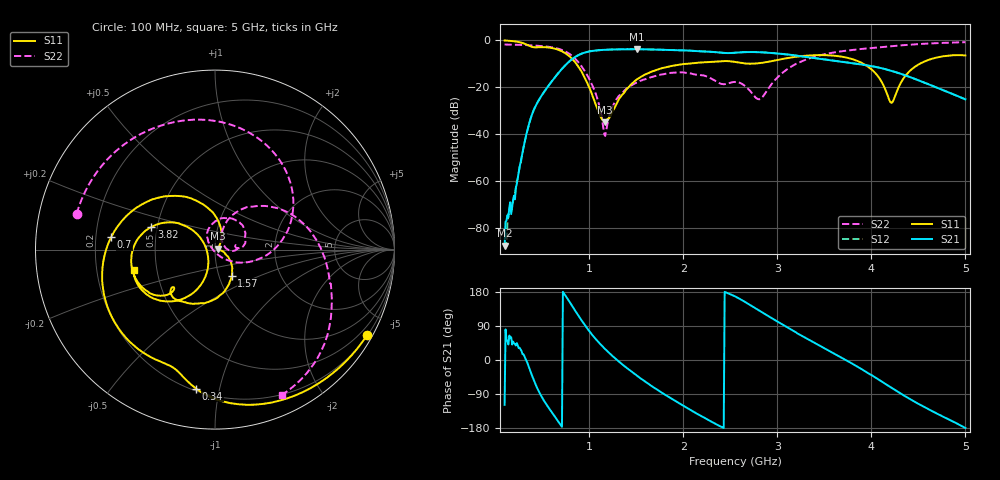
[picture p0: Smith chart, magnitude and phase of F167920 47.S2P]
!  2-Port S-parameters saved by WinCal
! VAR MeasName=S-Parameters (CALIBRATED_DATA) read from VNA (N5242A)
! VAR MeasDate=2016-11-22 9:57:49
! VAR NAME=F167920 47
! VAR FILENAME=F167920 47.S2P
! VAR DATE=2016-11-22 9:57:49
! VAR PHYS_PORTS=1,2
# Hz S DB R 50
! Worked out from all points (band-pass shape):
!   491 points, 100 MHz to 5 GHz, reference 50 ohm
!   highest |S21| = -3.95 dB at 1.51 GHz (marker M1); lowest = -87.6 dB at 100 MHz (marker M2)
!   |S21| within 3 dB of the highest: 863.3 MHz to 3.248 GHz (2.385 GHz wide, 116 % of centre)
!   lowest |S11| = -35.0 dB at 1.17 GHz (marker M3), VSWR 1.04, Z = 51.7 + j0.505 ohm
!   |S11| at or under -10 dB: 859.5 MHz to 2.083 GHz (1.223 GHz wide, 83.1 % of centre); 2.647 GHz to 2.787 GHz (140.3 MHz wide, 5.16 % of centre); 3.907 GHz to 4.523 GHz (616.1 MHz wide, 14.6 % of centre)
!   |S22| runs from -40.8 to -1.0 dB; largest |S21 - S12| = 0.0023
!   S11 on the Smith chart (normalised r, x): 100 MHz: 0.22, -3.82; 340 MHz: 0.21, -0.85; 700 MHz: 0.26, +0.06; 1.57 GHz: 1.15, -0.35; 3.82 GHz: 0.46, +0.14; 5 GHz: 0.37, -0.11
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1e8  -0.25 -29.3  -87.55 -118.4  -81.79 4.1  -1.98 165.5
1.9e8  -0.55 -55.1  -68.06 48.7  -68.67 36.1  -2.04 152.3
3.4e8  -2.14 -97.7  -38.80 -6.2  -38.84 -6.6  -2.24 129.1
4.5e8  -3.17 -116.6  -26.59 -75.9  -26.56 -75.8  -2.50 110.5
7e8  -4.69 173.0  -12.77 -172.7  -12.76 -172.7  -4.14 55.7
9.2e8  -13.60 93.6  -5.83 104.0  -5.83 104.0  -11.37 -9.1
1.06e9  -26.53 50.5  -4.57 57.9  -4.57 57.9  -21.92 -42.6
1.17e9  -34.98 15.9  -4.22 28.6  -4.22 28.6  -40.84 -145.2
1.29e9  -27.17 -12.5  -4.05 1.2  -4.05 1.2  -25.26 131.0
1.51e9  -16.70 -49.1  -3.95 -42.0  -3.96 -42.0  -18.10 104.9
1.57e9  -15.22 -57.1  -4.00 -52.7  -3.99 -52.6  -17.01 97.9
1.74e9  -12.43 -77.7  -4.17 -81.1  -4.17 -81.1  -14.94 77.2
2.13e9  -9.83 -110.7  -4.75 -139.7  -4.74 -139.7  -14.75 23.5
2.55e9  -9.39 -137.0  -5.48 167.9  -5.47 167.8  -17.89 7.8
2.82e9  -9.85 -135.7  -5.27 128.6  -5.26 128.5  -25.17 36.9
3.06e9  -8.08 -139.3  -6.02 92.9  -6.00 92.8  -13.84 64.4
3.37e9  -6.56 -159.1  -7.60 48.6  -7.57 48.4  -7.49 32.8
3.82e9  -8.49 160.4  -10.01 -13.0  -10.01 -13.2  -4.17 -5.7
4.05e9  -14.46 140.1  -11.53 -47.3  -11.54 -47.5  -3.26 -19.2
4.19e9  -25.46 166.5  -12.90 -69.5  -12.91 -69.7  -2.77 -26.7
4.5e9  -10.51 -119.8  -17.17 -115.7  -17.17 -116.0  -1.80 -42.6
5e9  -6.62 -166.1  -25.28 -179.5  -25.32 -179.8  -1.00 -65.1
